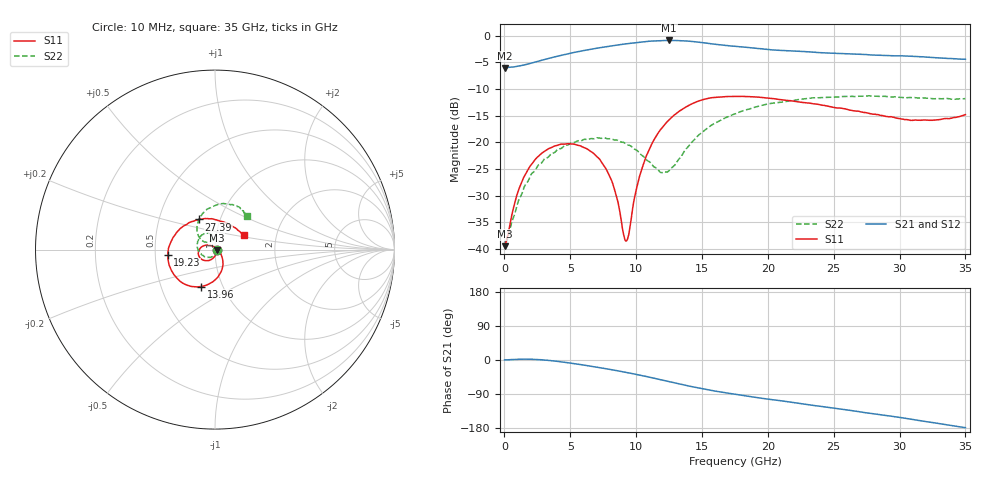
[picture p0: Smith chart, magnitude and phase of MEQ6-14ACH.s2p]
! MARKI MICROWAVE INC.
! Email:  support@markimicrowave.com  Phone:  408-778-4200
! Model Number:  MEQ6-14ACH  Date:  6/18
! Filename:		MEQ6-14ACH.S2P  Version: 1.0
! Description:  2-port S-parameter data for chip equalizer
! Features:		Low Insertion Loss, Excellent Return Loss
! Frequency Measured: 	10 MHz to 35 GHz
!S2P File: Measurements: S11, S21, S12, S22:
# Hz S  dB  R 50
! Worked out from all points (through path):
!   1601 points, 10 MHz to 35 GHz, reference 50 ohm
!   highest |S21| = -0.92 dB at 12.5 GHz (marker M1); lowest = -6.1 dB at 10 MHz (marker M2)
!   group delay of S21, straight-line fit = 15.6 ps
!   lowest |S11| = -39.5 dB at 10 MHz (marker M3), VSWR 1.02, Z = 51 - j0.379 ohm
!   |S11| at or under -10 dB: start of sweep to end of sweep
!   |S22| runs from -38.7 to -11.3 dB; largest |S21 - S12| = 0.011
!   S11 on the Smith chart (normalised r, x): 10 MHz: 1.02, -0.01; 13.96 GHz: 0.79, -0.34; 19.23 GHz: 0.58, -0.04; 27.39 GHz: 0.79, +0.28; 35 GHz: 1.37, +0.22
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1e7  -39.45 -20.4  -6.07 0.3  -5.93 -0.1  -38.69 -11.2
1.0597e9  -29.00 -89.8  -5.73 1.9  -5.73 1.9  -30.96 -88.1
2.218744e9  -23.59 -116.3  -5.04 1.7  -5.05 1.7  -25.57 -124.2
3.880769e9  -20.64 -145.3  -3.95 -3.0  -3.94 -3.1  -21.74 -163.7
5.848956e9  -20.76 -175.2  -2.89 -12.5  -2.89 -12.5  -19.71 160.2
7.117344e9  -22.91 164.8  -2.33 -19.5  -2.33 -19.5  -19.16 140.1
7.926488e9  -26.06 149.6  -2.02 -24.3  -2.02 -24.3  -19.33 127.2
8.451338e9  -29.69 135.7  -1.83 -27.6  -1.82 -27.5  -19.56 119.9
9.041794e9  -37.23 97.0  -1.61 -31.4  -1.61 -31.4  -20.02 112.9
9.260481e9  -38.43 51.7  -1.54 -32.8  -1.54 -32.8  -20.36 110.6
1.035392e10  -25.57 -44.5  -1.21 -40.5  -1.21 -40.4  -22.28 101.7
1.168791e10  -18.19 -72.7  -0.97 -50.7  -0.95 -50.5  -25.21 110.9
1.249706e10  -15.79 -87.4  -0.92 -56.9  -0.90 -56.9  -25.33 129.5
1.396226e10  -13.13 -110.8  -1.04 -68.4  -1.03 -68.3  -20.78 144.2
1.562429e10  -11.68 -134.9  -1.52 -79.9  -1.45 -79.8  -16.95 134.5
1.7505e10  -11.39 -156.6  -2.02 -90.3  -1.99 -90.5  -14.68 119.9
1.923263e10  -11.53 -173.3  -2.44 -99.5  -2.36 -99.5  -13.28 106.7
2.334396e10  -12.74 153.2  -3.10 -119.2  -3.04 -119.3  -11.68 80.7
2.738968e10  -14.42 118.0  -3.56 -139.0  -3.53 -139.0  -11.33 62.2
2.918291e10  -15.23 98.8  -3.77 -147.4  -3.74 -148.2  -11.45 55.5
3.239762e10  -15.86 59.1  -4.10 -164.6  -4.05 -164.5  -11.80 48.1
3.5e10  -14.81 25.7  -4.44 -178.5  -4.50 -178.6  -11.81 46.2
